(* Logix 5000 AddOnInstructionDefinition export OM_AZ_DDO; software revision 32.00 *)

ADD_ON_INSTRUCTION OM_AZ_DDO   (* revision 1.3, vendor ORIENTALMOTOR CO.,LTD. *)
// Revision note:
// Implicit message based on AZD-AEP,-CEP and -KEP.
// Help:
// Direct data operation(DDO) is a mode that allows rewriting of data and start of operation to be executed at the same time.
//  It is suitable to be used in frequently changed operation data such as the position (travel amount) and operating speed or to fine-tune the position.
// There are seven types of triggers to start operation at the same time as rewriting of data.
// -By changing one of the following items: Operation type, position, operating speed, starting/changing speed rate, stopping deceleration, and operating current. The six items are collectively rewritten.
// The direct data operation is executed by the TRIG of fixed I/O (IN).
// The condition to execute direct data operation can be selected from the following two types of parameters ON edge, or ON level by using the TRIG-MODE of fixed I/O (IN).
// - When executing "Set_Exe" the TRIG-MODE is set at ON level : The motor will start at the same time when the data of the trigger set in the "Direct data operation trigger setting" parameter is changed.
VAR_IN_OUT
   ImplicitMSGinput : INT[28]; {required}   // Implicit message Input (driver->scanner)
        [0]   // Remote I/O (R-OUT)
        [0].0   // R-OUT0
        [0].1   // R-OUT1
        [0].2   // R-OUT2
        [0].3   // R-OUT3
        [0].4   // R-OUT4
        [0].5   // R-OUT5
        [0].6   // R-OUT6
        [0].7   // R-OUT7
        [0].8   // R-OUT8
        [0].9   // R-OUT9
        [0].10   // R-OUT10
        [0].11   // R-OUT11
        [0].12   // R-OUT12
        [0].13   // R-OUT13
        [0].14   // R-OUT14
        [0].15   // R-OUT15
        [1]   // Operation data number selection_R
        [1].0   // M0_R
        [1].1   // M1_R
        [1].2   // M2_R
        [1].3   // M3_R
        [1].4   // M4_R
        [1].5   // M5_R
        [1].6   // M6_R
        [1].7   // M7_R
        [1].8   // Reserved
        [1].9   // Reserved
        [1].10   // Reserved
        [1].11   // Reserved
        [1].12   // Reserved
        [1].13   // Reserved
        [1].14   // Reserved
        [1].15   // Reserved
        [2]   // Fixed I/O (OUT)
        [2].0   // SEQ-BSY
        [2].1   // MOVE
        [2].2   // IN-POS
        [2].3   // START_R
        [2].4   // HOME-END
        [2].5   // READY
        [2].6   // DCMD-RDY
        [2].7   // ALM-A
        [2].8   // TRIG_R
        [2].9   // TRIG-MODE_R
        [2].10   // SET-ERR
        [2].11   // EXE-ERR
        [2].12   // DCMD-FULL
        [2].13   // STOP_R
        [2].14   // ETO-MON
        [2].15   // TLC
        [3]   // Present alarm
        [4]   // Feedback position (lower)
        [5]   // Feedback position (upper)
        [6]   // Feedback speed [Hz] (lower)
        [7]   // Feedback speed [Hz] (upper)
        [8]   // Command position (lower)
        [9]   // Command position (upper)
        [10]   // Torque monitor
        [11]   // CST operating current
        [12]   // Information (lower)
        [13]   // Information (upper)
        [14]   // Reserved
        [15]   // Read parameter ID_R
        [16]   // Read/write status
        [16].0   // Reserved
        [16].1   // Reserved
        [16].2   // Reserved
        [16].3   // Reserved
        [16].4   // Reserved
        [16].5   // Reserved
        [16].6   // Reserved
        [16].7   // RD-ERR
        [16].8   // WR-END
        [16].9   // SYS-BSY
        [16].10   // Reserved
        [16].11   // WR-SET-ERR
        [16].12   // WR-IF-ERR
        [16].13   // WR-NV-ERR
        [16].14   // WR-EXE-ERR
        [16].15   // WR-ERR
        [17]   // Write parameter ID_R
        [18]   // Read data (lower)
        [19]   // Read data (upper)
        [20]   // Assignable monitor 0 (lower)
        [21]   // Assignable monitor 0 (upper)
        [22]   // Assignable monitor 1 (lower)
        [23]   // Assignable monitor 1 (upper)
        [24]   // Assignable monitor 2 (lower)
        [25]   // Assignable monitor 2 (upper)
        [26]   // Assignable monitor 3 (lower)
        [27]   // Assignable monitor 3 (upper)
   ImplicitMSGoutput : INT[20]; {required}   // Implicit message Output (scanner->driver)
        [0]   // Remote I/O(R-IN)
        [0].0   // R-IN0
        [0].1   // R-IN1
        [0].2   // R-IN2
        [0].3   // R-IN3
        [0].4   // R-IN4
        [0].5   // R-IN5
        [0].6   // R-IN6
        [0].7   // R-IN7
        [0].8   // R-IN8
        [0].9   // R-IN9
        [0].10   // R-IN10
        [0].11   // R-IN11
        [0].12   // R-IN12
        [0].13   // R-IN13
        [0].14   // R-IN14
        [0].15   // R-IN15
        [1]   // Operation data number selection
        [1].0   // M0
        [1].1   // M1
        [1].2   // M2
        [1].3   // M3
        [1].4   // M4
        [1].5   // M5
        [1].6   // M6
        [1].7   // M7
        [1].8   // Reserved
        [1].9   // Reserved
        [1].10   // Reserved
        [1].11   // Reserved
        [1].12   // Reserved
        [1].13   // Reserved
        [1].14   // Reserved
        [1].15   // Reserved
        [2]   // Fixed I/O(IN)
        [2].0   // FW-JOG
        [2].1   // RV-JOG
        [2].2   // Reserved
        [2].3   // START
        [2].4   // ZHOME
        [2].5   // STOP
        [2].6   // FREE
        [2].7   // ALM-RST
        [2].8   // TRIG
        [2].9   // TRIG-MODE
        [2].10   // ETO-CLR
        [2].11   // Reserved
        [2].12   // FW-JOG-P
        [2].13   // RV-JOG-P
        [2].14   // FW-POS
        [2].15   // RV-POS
        [3]   // Direct data operation operation type
        [4]   // Direct data operation position (lower)
        [5]   // Direct data operation position (upper)
        [6]   // Direct data operation operating speed (lower)
        [7]   // Direct data operation operating speed (upper)
        [8]   // Direct data operation starting/changing rate (lower)
        [9]   // Direct data operation starting/changing rate (upper)
        [10]   // Direct data operation stopping deceleration (lower)
        [11]   // Direct data operation stopping deceleration (upper)
        [12]   // Direct data operation operating current
        [13]   // Direct data operation forwarding destination
        [14]   // Reserved
        [15]   // Read parameter ID
        [16]   // Write request
        [16].0   // WR-REQ
        [16].1   // Reserved
        [16].2   // Reserved
        [16].3   // Reserved
        [16].4   // Reserved
        [16].5   // Reserved
        [16].6   // Reserved
        [16].7   // Reserved
        [16].8   // Reserved
        [16].9   // Reserved
        [16].10   // Reserved
        [16].11   // Reserved
        [16].12   // Reserved
        [16].13   // Reserved
        [16].14   // Reserved
        [16].15   // Reserved
        [17]   // Write parameter ID
        [18]   // Write data (lower)
        [19]   // Write data (upper)
END_VAR
VAR_INPUT
   Set_Exe : BOOL; {visible}   // Execute AOI
   Set_OpeType : INT := 2; {visible}   // Direct data operation operation type
   Set_Position : DINT; {visible}   // Direct data operation position
   Set_Velocity : DINT := 1000; {visible}   // Direct data operation operating speed
   Set_Acceleration : DINT := 1000000; {visible}   // Direct data operation starting/changing rate
   Set_Deceleration : DINT := 1000000; {visible}   // Direct data operation stopping deceleration
   Set_Current : INT := 1000; {visible}   // Direct data operation operating current
   Set_Send : INT; {visible}   // Direct data operation forwarding destination
END_VAR
VAR_OUTPUT
   Sts_Busy : BOOL; {access Read Only, visible}   // Executing status in AOI
   Sts_Err : BOOL; {access Read Only, visible}   // Error status in AOI
   Sts_Done : BOOL; {access Read Only, visible}   // Complete status in AOI
   Read_Present_alarm : INT; {access Read Only, visible}   // Alarm code monitor[Hex]
   Read_Command_position : DINT; {access Read Only, visible}   // Command position monitor[step]
   Read_Feedback_position : DINT; {access Read Only, visible}   // Feedback position monitor[step]
   Read_Torque_monitor : INT; {access Read Only, visible}   // Torque monitor as a percentage of the maximum holding torque(1=0.1%)
   Read_Cumulative_load_monitor : DINT; {access Read Only, visible}   // Cumulative load monitor
END_VAR
VAR
   flag_Exe : BOOL; {access None}
   flag_End : BOOL; {access None}
   flag_Ini : BOOL; {access None}
   flag_Ready : BOOL; {access None}
   FixedIO_OUT : INT;   // Fixed I/O(OUT)
        .0   // SEQ-BSY
        .1   // MOVE
        .2   // IN-POS
        .3   // START_R
        .4   // HOME-END
        .5   // READY
        .6   // DCMD-RDY
        .7   // ALM-A
        .8   // TRIG_R
        .9   // TRIG-MODE_R
        .10   // SET-ERR
        .11   // EXE-ERR
        .12   // DCMD-FULL
        .13   // STOP_R
        .14   // ETO-MON
        .15   // TLC
   flag_Exe3 : BOOL; {access None}
   flag_Exe2 : BOOL; {access None}
END_VAR

ROUTINE Logic   (* ladder *)
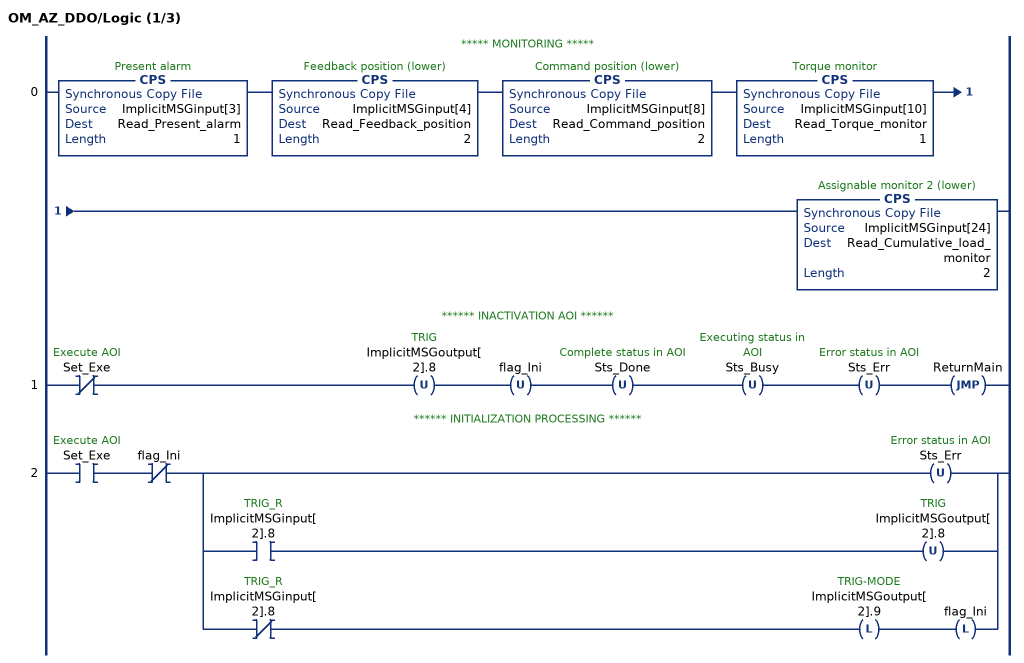
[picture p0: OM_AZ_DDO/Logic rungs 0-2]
   // ***** MONITORING *****
   0: CPS(ImplicitMSGinput[3],Read_Present_alarm,1)CPS(ImplicitMSGinput[4],Read_Feedback_position,2)CPS(ImplicitMSGinput[8],Read_Command_position,2)CPS(ImplicitMSGinput[10],Read_Torque_monitor,1)CPS(ImplicitMSGinput[24],Read_Cumulative_load_monitor,2);
   // ****** INACTIVATION AOI ******
   1: XIO(Set_Exe)OTU(ImplicitMSGoutput[2].8)OTU(flag_Ini)OTU(Sts_Done)OTU(Sts_Busy)OTU(Sts_Err)JMP(ReturnMain);
   // ****** INITIALIZATION PROCESSING ******
   2: XIC(Set_Exe)XIO(flag_Ini)[OTU(Sts_Err) ,[XIC(ImplicitMSGinput[2].8) OTU(ImplicitMSGoutput[2].8) ,XIO(ImplicitMSGinput[2].8) OTL(ImplicitMSGoutput[2].9) OTL(flag_Ini) ] ];
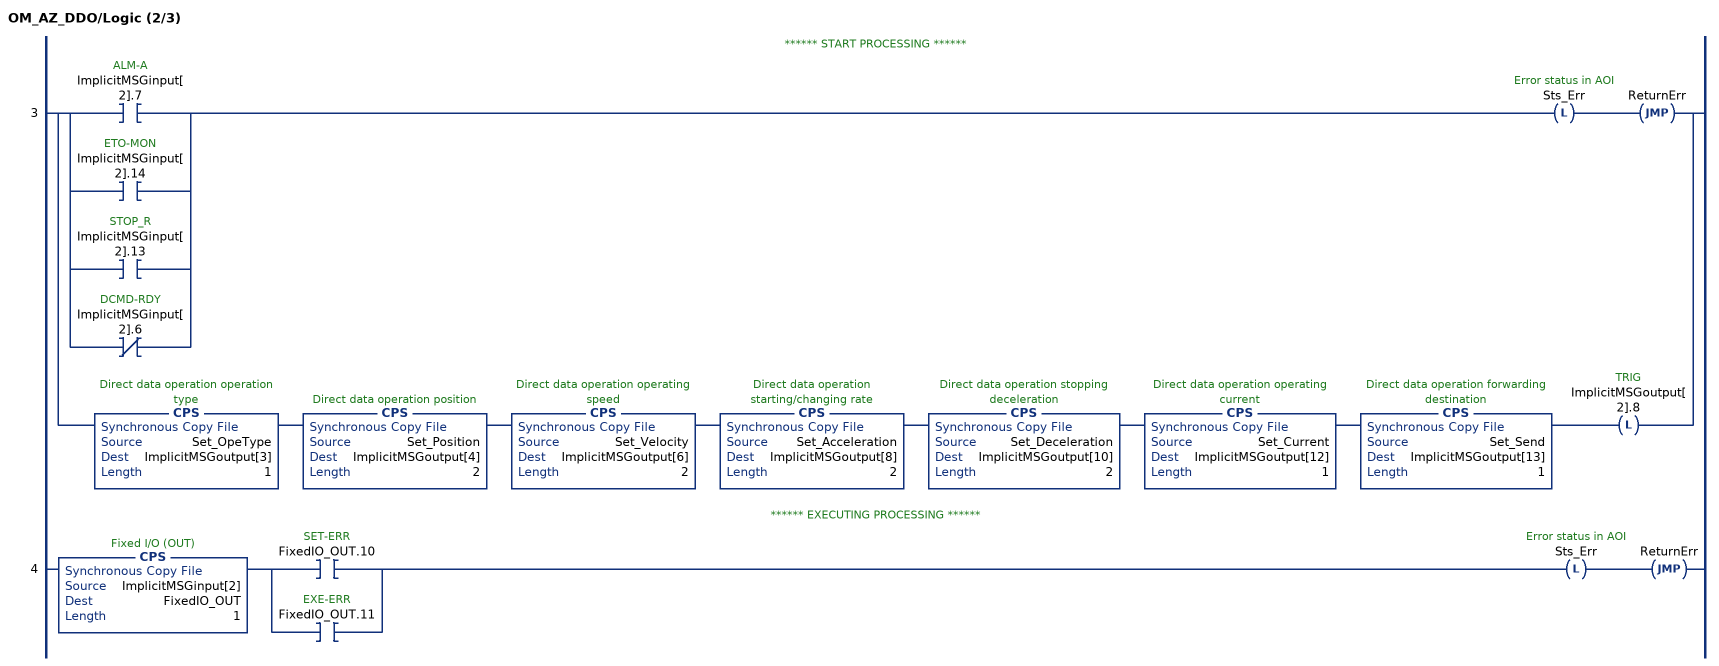
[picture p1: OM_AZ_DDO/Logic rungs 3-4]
   // ****** START PROCESSING ******
   3: [[XIC(ImplicitMSGinput[2].7) ,XIC(ImplicitMSGinput[2].14) ,[XIC(ImplicitMSGinput[2].13) ,XIO(ImplicitMSGinput[2].6) ] ] OTL(Sts_Err) JMP(ReturnErr) ,CPS(Set_OpeType,ImplicitMSGoutput[3],1) CPS(Set_Position,ImplicitMSGoutput[4],2) CPS(Set_Velocity,ImplicitMSGoutput[6],2) CPS(Set_Acceleration,ImplicitMSGoutput[8],2) CPS(Set_Deceleration,ImplicitMSGoutput[10],2) CPS(Set_Current,ImplicitMSGoutput[12],1) CPS(Set_Send,ImplicitMSGoutput[13],1) OTL(ImplicitMSGoutput[2].8) ];
   // ****** EXECUTING PROCESSING ******
   4: CPS(ImplicitMSGinput[2],FixedIO_OUT,1)[XIC(FixedIO_OUT.10) ,XIC(FixedIO_OUT.11) ]OTL(Sts_Err)JMP(ReturnErr);
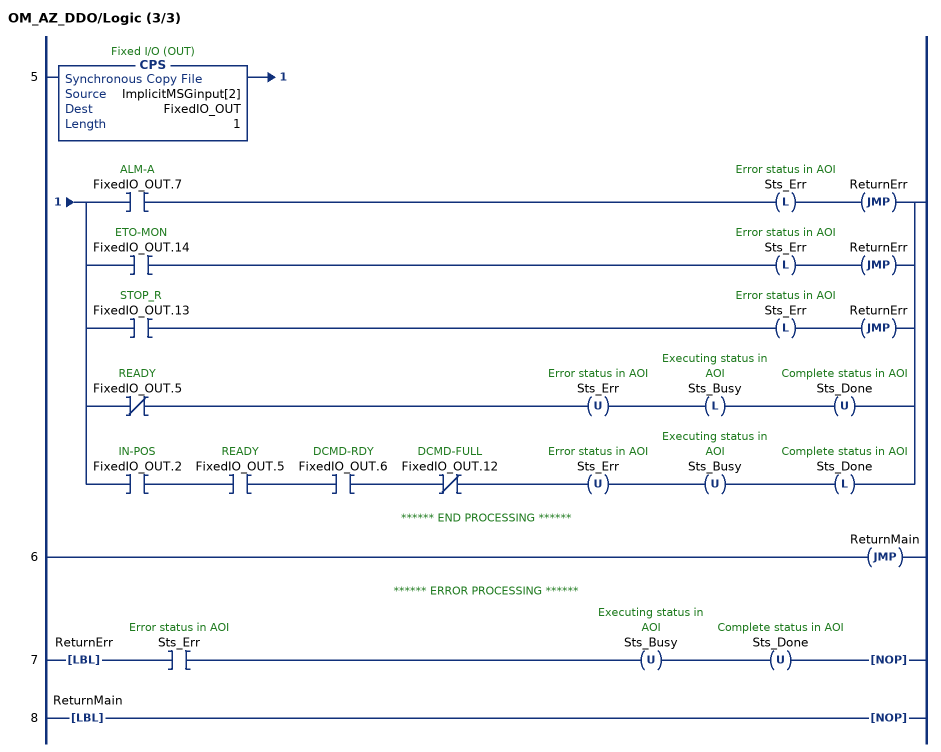
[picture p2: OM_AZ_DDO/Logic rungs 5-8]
   5: CPS(ImplicitMSGinput[2],FixedIO_OUT,1)[XIC(FixedIO_OUT.7) OTL(Sts_Err) JMP(ReturnErr) ,[XIC(FixedIO_OUT.14) OTL(Sts_Err) JMP(ReturnErr) ,XIC(FixedIO_OUT.13) OTL(Sts_Err) JMP(ReturnErr) ,XIO(FixedIO_OUT.5) OTU(Sts_Err) OTL(Sts_Busy) OTU(Sts_Done) ,XIC(FixedIO_OUT.2) XIC(FixedIO_OUT.5) XIC(FixedIO_OUT.6) XIO(FixedIO_OUT.12) OTU(Sts_Err) OTU(Sts_Busy) OTL(Sts_Done) ] ];
   // ****** END PROCESSING ******
   6: JMP(ReturnMain);
   // ****** ERROR PROCESSING ******
   7: LBL(ReturnErr)XIC(Sts_Err)OTU(Sts_Busy)OTU(Sts_Done)NOP();
   8: LBL(ReturnMain)NOP();
END_ROUTINE
END_ADD_ON_INSTRUCTION
